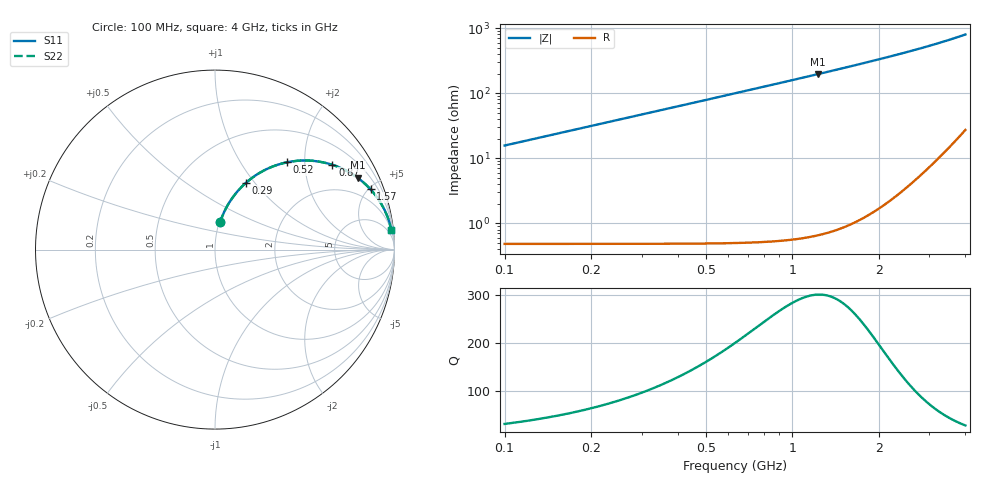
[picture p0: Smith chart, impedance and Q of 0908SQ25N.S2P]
! Coilcraft 0908SQ-25N Air Core Inductor
! 15 June 2010
# MHZ S MA R 50
!Freq  MagS11  AngS11  MagS21  AngS21  MagS12  AngS12  MagS22  AngS22
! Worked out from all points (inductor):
!   391 points, 100 MHz to 4 GHz, reference 50 ohm
!   read as one part in series: L = 24.9 nH near 110 MHz
!   highest Q = 301 at 1.23 GHz (marker M1), where L = 25.4 nH
!   S11 on the Smith chart (normalised r, x): 100 MHz: 1.01, +0.31; 290 MHz: 1.01, +0.91; 520 MHz: 1.01, +1.63; 870 MHz: 1.02, +2.76; 1.57 GHz: 1.05, +5.15; 4 GHz: 2, +18
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100  0.1538 79.4  0.9834 -8.9  0.9834 -8.9  0.1538 79.4
120  0.1836 77.9  0.9783 -10.6  0.9783 -10.6  0.1836 77.9
140  0.2129 76.4  0.9724 -12.3  0.9724 -12.3  0.2129 76.4
180  0.2697 73.3  0.9583 -15.7  0.9583 -15.7  0.2697 73.3
230  0.337 69.5  0.937 -19.7  0.937 -19.7  0.3371 69.5
290  0.4115 65.0  0.907 -24.4  0.907 -24.4  0.4116 65.0
340  0.468 61.5  0.8795 -28.0  0.8795 -28.0  0.4681 61.5
390  0.5194 58.2  0.8504 -31.4  0.8504 -31.4  0.5194 58.2
450  0.5744 54.5  0.8146 -35.1  0.8146 -35.1  0.5745 54.5
520  0.6302 50.5  0.7727 -39.2  0.7727 -39.2  0.6302 50.5
630  0.7018 45.0  0.7089 -44.7  0.7089 -44.7  0.7018 45.0
750  0.7616 40.0  0.6448 -49.7  0.6448 -49.7  0.7616 40.0
870  0.807 35.8  0.5874 -54.0  0.5874 -54.0  0.8071 35.8
1040  0.8539 31.0  0.5175 -58.8  0.5175 -58.8  0.8539 31.0
1230  0.8899 26.7  0.4533 -63.1  0.4533 -63.1  0.8899 26.7
1400  0.9126 23.7  0.4058 -66.1  0.4058 -66.1  0.9126 23.7
1570  0.9293 21.2  0.3659 -68.6  0.3659 -68.6  0.9293 21.2
1790  0.945 18.5  0.3229 -71.3  0.3229 -71.3  0.9451 18.5
2050  0.958 16.0  0.2817 -73.7  0.2817 -73.7  0.958 16.0
2700  0.976 11.5  0.2082 -77.9  0.2082 -77.9  0.976 11.5
3350  0.9842 8.5  0.1591 -80.4  0.1591 -80.4  0.9842 8.5
4000  0.9881 6.3  0.1237 -81.7  0.1237 -81.7  0.9881 6.3
